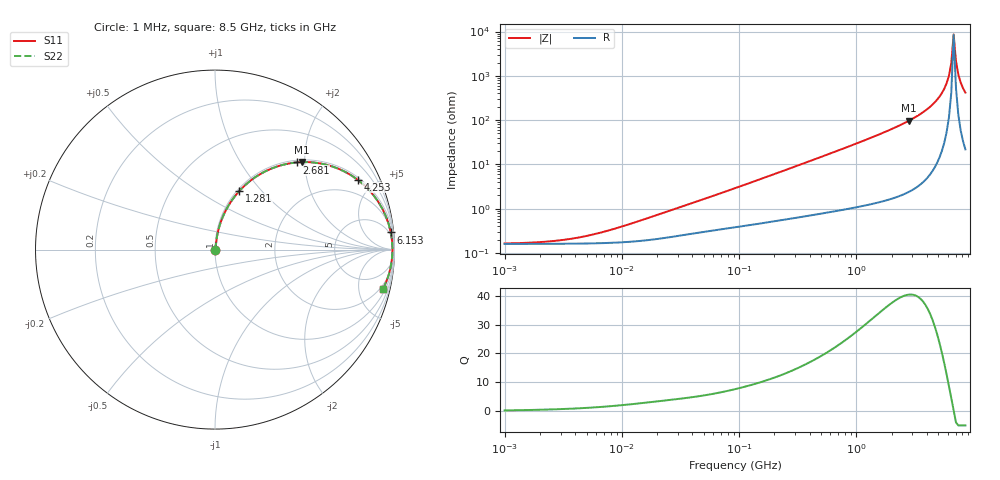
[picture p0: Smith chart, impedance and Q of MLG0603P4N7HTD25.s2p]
! S-Parameter Data Generated by TDK Corporation
! Copyright(C) 2025 TDK Corporation.
! All Rights Reserved.
! TDK P/N: MLG0603P4N7HTD25 (SMD / SMT Inductor (Coil))
! Property: L=4.7nH at 500MHz
! Size(LxWxT): 0.6x0.3x0.3mm
! Model Type: s2p (Touchstone File Format Version 1.0)
! Frequency: DC=Yes Start=1MHz Stop=8500MHz 198points Log-sweep
! Model Generated on Feb. 6, 2025
! Terms and conditions regarding TDK Simulation Models:
! 1)This simulation model is being provided solely for informational
!  purposes. Please refer to the specifications of the products in
!  terms of detailed characteristics of such products.
! 2)In no event shall TDK Corporation of any of its subsidiaries be
!  liable for any loss or damage arising, directly or indirectly,
!  from any information contained in this simulation model, including,
!  but not limited to loss or damages arising from any inaccuracies,
!  omissions or errors in connection with such information.
! 3)Any and all copyrights on this simulation model are owned by
!  TDK Corporation.  Duplication or redistribution of this simulation
!  model without prior written permission from TDK Corporation
!  is prohibited.
! 4)This simulation model is subject to any modification or change
!  without any prior notice.
! 5)Neither TDK Corporation nor any of its subsidiaries shall make any
!  warranty, express or implied, including but not limited to the
!  correctness, implied warranties of merchantability and fitness for
!  a particular purpose with respect to this simulation models.
! 6)The use of this simulation model shall be deemed to have consented
!  to the terms and conditions hereof.
! Port Assignments:
!  1 ---@@@--- 2
! Applicable Conditions:
!  Temperature = 25 degC
!  DC Bias Current = 0 A
!  Small Signal Operation
# Hz S MA R 50
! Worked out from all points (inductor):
!   197 points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, 1 MHz to 8.5 GHz, reference 50 ohm
!   read as one part in series: L = 5.49 nH near 17.5 MHz
!   highest Q = 40.4 at 2.807 GHz (marker M1), where L = 5.51 nH
!   self-resonance near 6.748 GHz
!   S11 on the Smith chart (normalised r, x): 1 MHz: 1.00, +0.00; 1.281 GHz: 1.02, +0.77; 2.681 GHz: 1.05, +1.82; 4.253 GHz: 1.12, +4.01; 6.153 GHz: 3, +20; 8.5 GHz: 1.44, -8.36
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1000000  0.001639 12.6  0.9984 -0.0  0.9984 -0.0  0.001639 12.6
2403882  0.001823 28.2  0.9984 -0.0  0.9984 -0.0  0.001823 28.2
4587603  0.002313 45.1  0.9984 -0.1  0.9984 -0.1  0.002313 45.1
8360083  0.003426 60.1  0.9983 -0.2  0.9983 -0.2  0.003426 60.1
2.10461e7  0.007556 73.4  0.9979 -0.4  0.9979 -0.4  0.007556 73.4
9.219544e7  0.02892 80.9  0.9958 -1.6  0.9958 -1.6  0.02892 80.9
4.229561e8  0.1236 79.6  0.9853 -7.1  0.9853 -7.1  0.1236 79.6
1.280704e9  0.3545 67.4  0.9237 -20.8  0.9237 -20.8  0.3545 67.4
1.940355e9  0.5133 57.6  0.8445 -30.9  0.8445 -30.9  0.5133 57.6
2.680511e9  0.6653 46.9  0.7302 -41.7  0.7302 -41.7  0.6653 46.9
2.80715e9  0.6883 45.1  0.7086 -43.5  0.7086 -43.5  0.6883 45.1
3.535948e9  0.8022 35.2  0.5768 -53.3  0.5768 -53.3  0.8022 35.2
4.253027e9  0.8847 26.1  0.4406 -62.2  0.4406 -62.2  0.8847 26.1
5.357206e9  0.9605 13.6  0.2348 -73.6  0.2348 -73.6  0.9605 13.6
5.87536e9  0.9784 8.3  0.1441 -77.3  0.1441 -77.3  0.9784 8.3
6.152938e9  0.9841 5.6  0.09774 -77.9  0.09774 -77.9  0.9841 5.6
6.44363e9  0.9876 2.9  0.0513 -74.6  0.0513 -74.6  0.9876 2.9
6.748056e9  0.9889 0.2  0.01149 -14.0  0.01149 -14.0  0.9889 0.2
7.066863e9  0.9878 -2.6  0.04588 73.3  0.04588 73.3  0.9878 -2.6
7.400733e9  0.9845 -5.3  0.09228 77.7  0.09228 77.7  0.9845 -5.3
7.750377e9  0.9789 -7.9  0.1387 77.3  0.1387 77.3  0.9789 -7.9
8.5e9  0.9613 -13.3  0.2298 73.7  0.2298 73.7  0.9613 -13.3
